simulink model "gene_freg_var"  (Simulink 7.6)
settings: Solver=ode14x  StartTime=0.0  StopTime=200  RelTol=1e-3
InitFcn:
  | clc, close all
  | C=0.1e-3;
  | R=1e3;
StopFcn:
  | close all, clc
  | load gene_freg_var.mat
  | plot(x(1,:),x(2,:))
  | title('Générateur de créneaux à fréquence variable')
  | xlabel('temps')
  | grid
undefined symbols (not defined in the file or in its folder): sigbuilder_block
libraries: fl_lib x10, nesl_utility x3, elec_lib x1

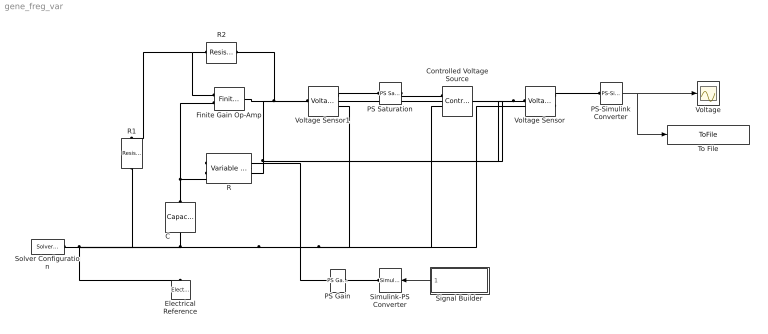
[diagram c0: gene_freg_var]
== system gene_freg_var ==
  C : fl_lib/Electrical/Electrical Elements/Capacitor  DialogController=NetworkEngine.DynNeDlgSource  SystemSampleTime=-1  c=C F  v0=1e-6 V  r=0 Ohm  g=0 1/Ohm  i_Log=off  v_Log=off  vc_Log=off  LocalVarNames=|i|v|vc  LocalVarDescs=|i|v|Internal variable for voltage across capacitor term  LocalVarLogging=[0 0 0]
  Controlled Voltage Source : fl_lib/Electrical/Electrical Sources/Controlled Voltage Source  DialogController=NetworkEngine.DynNeDlgSource  SystemSampleTime=-1  i_Log=off  v_Log=off  LocalVarNames=|i|v  LocalVarDescs=|i|v  LocalVarLogging=[0 0]
  Electrical Reference : fl_lib/Electrical/Electrical Elements/Electrical Reference  DialogController=NetworkEngine.DynNeDlgSource  SystemSampleTime=-1  i_Log=off  LocalVarNames=|i  LocalVarDescs=|i  LocalVarLogging=[]
  Finite Gain Op-Amp : elec_lib/Integrated Circuits/Finite Gain Op-Amp  DialogController=NetworkEngine.DynNeDlgSource  SystemSampleTime=-1  A=1000  Rin=1e+06 Ohm  Rout=100 Ohm  Vmin=-15 V  Vmax=15 V  LocalVarNames=|power  LocalVarDescs=|Dissipated power (W)  LocalVarLogging=0
  PS Gain : fl_lib/Physical Signals/Functions/PS Gain  DialogController=NetworkEngine.DynNeDlgSource  SystemSampleTime=-1  gain=1e4  LocalVarLogging=[]
  PS Saturation : fl_lib/Physical Signals/Nonlinear Operators/PS Saturation  DialogController=NetworkEngine.DynNeDlgSource  SystemSampleTime=-1  upper_limit=12  lower_limit=-12  LocalVarLogging=[]
  PS-Simulink Converter : nesl_utility/PS-Simulink Converter  DialogController=NetworkEngine.DynNeUtilDlgSource  SystemSampleTime=-1  PhysicalDomain=network_engine_domain  LeftPortType=input  RightPortType=output  SubClassName=ps_output  Unit=1  AffineConversion=off
  R : fl_lib/Electrical/Electrical Elements/Variable Resistor  DialogController=NetworkEngine.DynNeDlgSource  SystemSampleTime=-1  Rmin=0 Ohm  i_Log=off  v_Log=off  LocalVarNames=|i|v  LocalVarDescs=|i|v  LocalVarLogging=[0 0]
  R1 : fl_lib/Electrical/Electrical Elements/Resistor  DialogController=NetworkEngine.DynNeDlgSource  SystemSampleTime=-1  R=10 kOhm  i_Log=off  v_Log=off  LocalVarNames=|current|voltage|power  LocalVarDescs=|Resistor current (A)|Voltage across resistor (V)|Power (W)  LocalVarLogging=[0 0 0]
  R2 : fl_lib/Electrical/Electrical Elements/Resistor  DialogController=NetworkEngine.DynNeDlgSource  SystemSampleTime=-1  R=10 kOhm  i_Log=off  v_Log=off  LocalVarNames=|current|voltage|power  LocalVarDescs=|Resistor current (A)|Voltage across resistor (V)|Power (W)  LocalVarLogging=[0 0 0]
  Signal Builder : Subsystem  Tag=STV Subsys  LoadFcn=sigbuilder_block('load',[496.5 -36.75 550.5 399.75 ]);  StartFcn=sigbuilder_block('start');  StopFcn=sigbuilder_block('stop');  ClipboardFcn=sigbuilder_block('clipboard');
  Simulink-PS Converter : nesl_utility/Simulink-PS Converter  DialogController=NetworkEngine.DynNeUtilDlgSource  SystemSampleTime=-1  PhysicalDomain=network_engine_domain  LeftPortType=input  RightPortType=output  SubClassName=ps_input  Unit=1  AffineConversion=off  InputFilterTimeConstant=.001  UdotUserProvided=0
  Solver Configuration : nesl_utility/Solver Configuration  DialogController=NetworkEngine.DynNeUtilDlgSource  SystemSampleTime=-1  PhysicalDomain=network_engine_domain  LeftPortType=input  RightPortType=generic  SubClassName=solver  Accelerate=off  Profile=off  ResidualTolerance=1e-9  MaxNonlinIter=12  MaxModeIter=2  DoFixedCost=off  UseLocalSampling=off  DoDC=off  LinearAlgebra=Sparse  LocalSolverSampleTime=.001  LocalSolverChoice=NE_BACKWARD_EULER_ADVANCER  UseLocalSolver=off
  To File : ToFile  Filename=gene_freg_var  MatrixName=x
  Voltage : Scope
  Voltage Sensor : fl_lib/Electrical/Electrical Sensors/Voltage Sensor  DialogController=NetworkEngine.DynNeDlgSource  SystemSampleTime=-1  i1_Log=off  v1_Log=off  LocalVarNames=|i1|v1  LocalVarDescs=|i1|v1  LocalVarLogging=[]
  Voltage Sensor1 : fl_lib/Electrical/Electrical Sensors/Voltage Sensor  DialogController=NetworkEngine.DynNeDlgSource  SystemSampleTime=-1  i1_Log=off  v1_Log=off  LocalVarNames=|i1|v1  LocalVarDescs=|i1|v1  LocalVarLogging=[]
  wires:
  PS-Simulink Converter/1 -> Voltage/1, To File/1
  Signal Builder/1(Signal 2) -> Simulink-PS Converter/1
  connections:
  R/LConn2 -- Voltage Sensor/LConn1 -- Controlled Voltage Source/LConn1
  C/LConn1 -- Finite Gain Op-Amp/LConn2 -- R/RConn1
  Electrical Reference/LConn1 -- Voltage Sensor/RConn2 -- Controlled Voltage Source/RConn2 -- Voltage Sensor1/RConn2 -- C/RConn1 -- Solver Configuration/RConn1 -- R1/LConn1
  R2/LConn1 -- R1/RConn1 -- Finite Gain Op-Amp/LConn1
  Voltage Sensor/RConn1 -- PS-Simulink Converter/LConn1
  Voltage Sensor1/LConn1 -- R2/RConn1 -- Finite Gain Op-Amp/RConn1
  PS Saturation/RConn1 -- Controlled Voltage Source/RConn1
  Voltage Sensor1/RConn1 -- PS Saturation/LConn1
  Simulink-PS Converter/RConn1 -- PS Gain/LConn1
  PS Gain/RConn1 -- R/LConn1

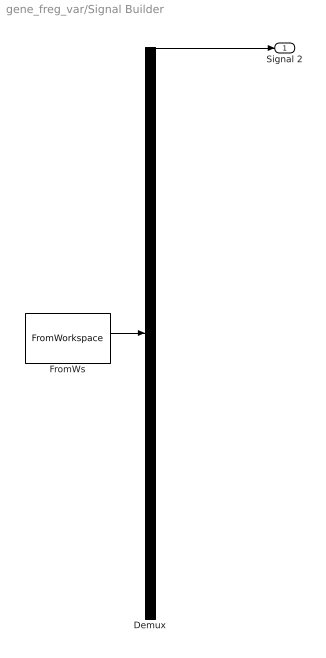
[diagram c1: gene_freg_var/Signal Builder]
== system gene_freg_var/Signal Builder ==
  Demux : Demux  Tag=STV Demux  Outputs=1
  FromWs : FromWorkspace  Tag=STV FromWs  VariableName=tuvar  SampleTime=0  SigBuilderData=DataTag0  VnvData=DataTag1
  Signal 2 : Outport  Tag=STV Outport
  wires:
  FromWs/1 -> Demux/1
  Demux/1 -> Signal 2/1
